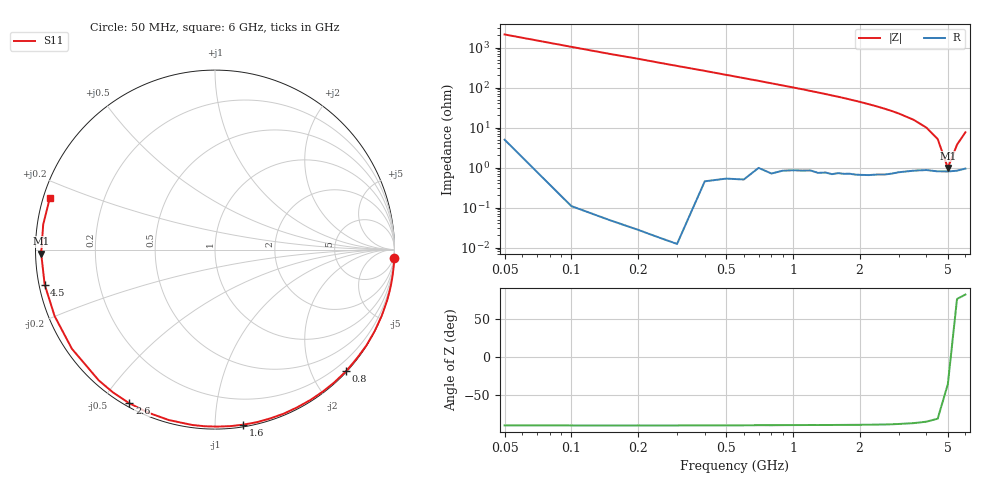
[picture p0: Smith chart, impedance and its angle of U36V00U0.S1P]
! SIEMENS Discrete & RF Semiconductors
! BBY53-02W
! Si Tuning Diode in SCD-80
! VR = 6 V
! S-Parameters:  September  1997
# GHz  S  MA  R  50
!  f  S11
! GHz  MAG  ANG
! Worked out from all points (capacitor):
!   34 points, 50 MHz to 6 GHz, reference 50 ohm
!   read as one part to ground: C = 1.53 pF near 50 MHz
!   lowest |Z| = 978 mohm at 5 GHz (marker M1)
!   series resonance near 5.068 GHz, so ESL is about 650 pH
!   S11 on the Smith chart (normalised r, x): 50 MHz: 0, -42; 800 MHz: 0.01, -2.55; 1.6 GHz: 0.01, -1.17; 2.6 GHz: 0.01, -0.59; 4.5 GHz: 0.02, -0.10; 6 GHz: 0.02, +0.15
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0.05  0.9999 -2.7
0.2  1 -10.9
0.3  1 -16.4
0.4  0.9994 -21.7
0.5  0.9988 -27.1
0.6  0.9984 -32.4
0.8  0.9962 -42.8
0.9  0.9945 -48.0
1  0.9933 -52.8
1.1  0.9922 -57.7
1.2  0.9909 -62.6
1.3  0.991 -67.3
1.4  0.9897 -72.0
1.5  0.9896 -76.5
1.6  0.9879 -80.8
1.8  0.9862 -89.4
2  0.9853 -97.4
2.2  0.9838 -105.1
2.4  0.9817 -112.3
2.6  0.9803 -119.1
2.8  0.9779 -125.5
3  0.975 -131.6
3.5  0.9701 -145.3
4  0.9673 -157.5
4.5  0.9688 -168.4
5  0.9686 -178.7
5.5  0.9674 171.7
6  0.9639 162.8
